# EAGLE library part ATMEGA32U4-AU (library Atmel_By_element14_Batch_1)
8-bit Microcontroller with ISP Flash and USB Controller
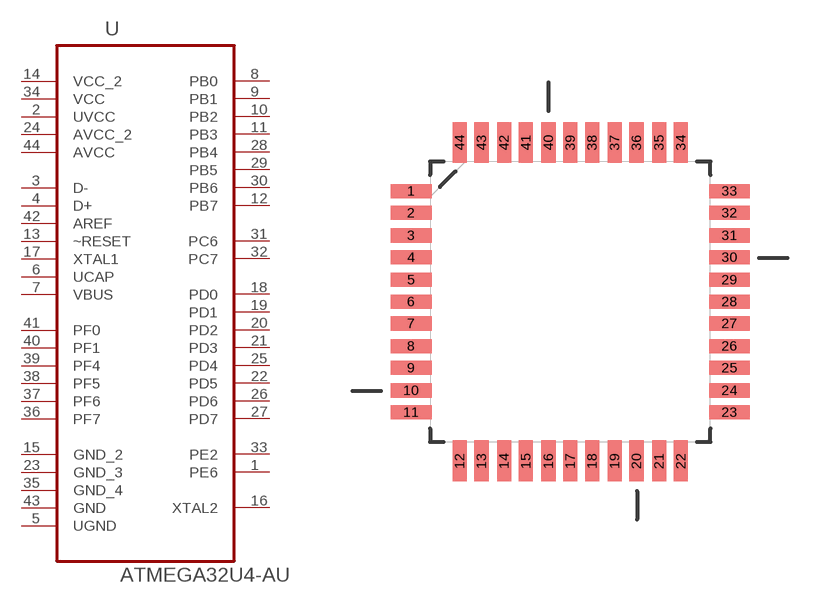
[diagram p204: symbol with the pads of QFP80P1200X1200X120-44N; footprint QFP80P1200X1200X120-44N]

Designator prefix U

## ATMEGA32U4-AU (MPN: ATMEGA32U4-AU; OC_FARNELL: 1748525; OC_NEWARK: 26R5633; PACKAGE: TQFP-44; SUPPLIER: Atmel)  [QFP80P1200X1200X120-44N]
1  PE6
2  UVCC  pwr
3  D-  pas
4  D+  pas
5  UGND  pas
6  UCAP  pwr
7  VBUS  in
8  PB0
9  PB1
10  PB2
11  PB3
12  PB7
13  ~RESET  in
14  VCC_2  pwr
15  GND_2  pas
16  XTAL2  out
17  XTAL1  in
18  PD0
19  PD1
20  PD2
21  PD3
22  PD5
23  GND_3  pas
24  AVCC_2  pwr
25  PD4
26  PD6
27  PD7
28  PB4
29  PB5
30  PB6
31  PC6
32  PC7
33  PE2
34  VCC  pwr
35  GND_4  pas
36  PF7
37  PF6
38  PF5
39  PF4
40  PF1
41  PF0
42  AREF  in
43  GND  pas
44  AVCC  pwr

## Footprint QFP80P1200X1200X120-44N (pad centres in mm)
smd 1.473 x 0.508: 1 -5.74,3.988; 2 -5.74,3.2; 3 -5.74,2.388; 4 -5.74,1.6; 5 -5.74,0.787; 6 -5.74,0; 7 -5.74,-0.787; 8 -5.74,-1.6; 9 -5.74,-2.388; 10 -5.74,-3.2; 11 -5.74,-3.988; 23 5.74,-3.988; 24 5.74,-3.2; 25 5.74,-2.388; 26 5.74,-1.6; 27 5.74,-0.787; 28 5.74,0; 29 5.74,0.787; 30 5.74,1.6; 31 5.74,2.388; 32 5.74,3.2; 33 5.74,3.988
smd 0.508 x 1.473: 12 -3.988,-5.74; 13 -3.2,-5.74; 14 -2.388,-5.74; 15 -1.6,-5.74; 16 -0.787,-5.74; 17 0,-5.74; 18 0.787,-5.74; 19 1.6,-5.74; 20 2.388,-5.74; 21 3.2,-5.74; 22 3.988,-5.74; 34 3.988,5.74; 35 3.2,5.74; 36 2.388,5.74; 37 1.6,5.74; 38 0.787,5.74; 39 0,5.74; 40 -0.787,5.74; 41 -1.6,5.74; 42 -2.388,5.74; 43 -3.2,5.74; 44 -3.988,5.74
